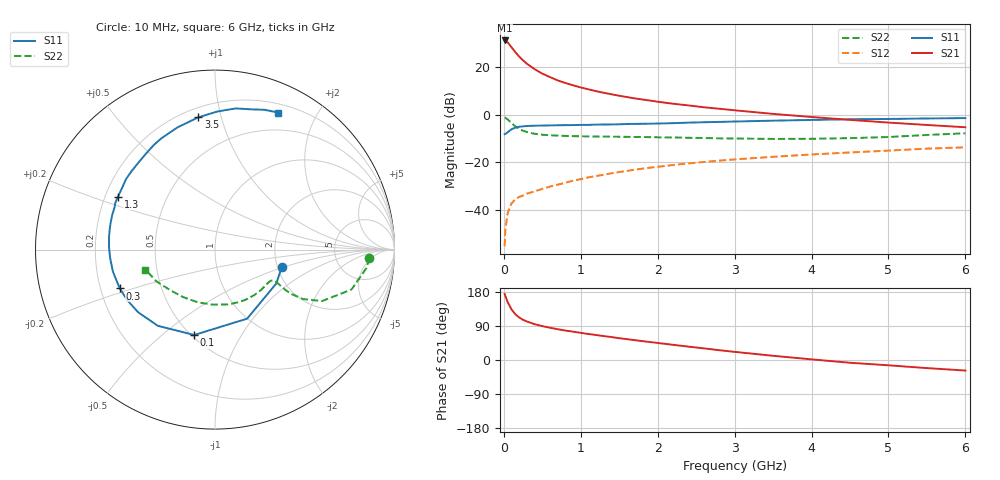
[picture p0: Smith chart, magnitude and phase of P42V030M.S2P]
! SIEMENS Small Signal Semiconductors
! BFP182
! Si NPN RF Bipolar Junction Transistor in SOT143
! VCE = 2 V  IC = 30 mA
! Common Emitter S-Parameters:  March  1996
# GHz  S  MA  R  50
!  f  S11  S21  S12  S22
! GHz  MAG  ANG  MAG  ANG  MAG  ANG  MAG  ANG
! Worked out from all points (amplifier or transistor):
!   36 points, 10 MHz to 6 GHz, reference 50 ohm
!   highest |S21| = 31.2 dB at 10 MHz (marker M1)
!   |S21| within 3 dB of that: start of sweep to 102.9 MHz
!   unconditionally stable (mu >= 1): start of sweep to 17.58 MHz; 309.4 MHz to end of sweep
!   at 250 MHz: K = 0.90, MSG = 28.4 dB, |S12| = -34.1 dB
!   at 1.4 GHz: K = 1.63, MAG = 12.0 dB, |S12| = -24.7 dB
!   at 6 GHz: K = 1.15, MAG = 1.8 dB, |S12| = -13.8 dB
!   S11 on the Smith chart (normalised r, x): 10 MHz: 2.11, -0.48; 100 MHz: 0.52, -0.65; 300 MHz: 0.28, -0.18; 1.3 GHz: 0.25, +0.24; 3.5 GHz: 0.26, +0.85; 6 GHz: 0.29, +1.52
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0.01  0.3846 -14.6  36.18 174.2  0.0017 75.7  0.8603 -3.1
0.02  0.3903 -28.9  35.97 168.9  0.0038 73.8  0.8513 -6.8
0.05  0.4244 -65.1  33.08 152.7  0.0085 71.5  0.7923 -16.3
0.1  0.4897 -103.7  25.97 133.4  0.0135 54.7  0.6617 -25.7
0.15  0.5308 -126.9  20.45 120.6  0.0166 48.1  0.5628 -29.3
0.2  0.5528 -140.9  16.56 112.1  0.0185 46.9  0.4966 -30.1
0.25  0.5647 -150.4  13.76 106.1  0.0198 47.6  0.4551 -29.9
0.3  0.5732 -157.8  11.72 101.6  0.0217 47.6  0.4274 -29.1
0.4  0.582 -168.0  8.989 94.5  0.0241 49.6  0.3936 -28.1
0.5  0.5859 -175.2  7.256 89.4  0.0273 50.9  0.3756 -27.8
0.6  0.5906 178.9  6.129 85.1  0.0305 53.5  0.3665 -28.0
0.7  0.5946 173.5  5.224 81.2  0.0334 55.4  0.3595 -28.7
0.8  0.5973 169.3  4.61 77.7  0.0367 55.8  0.3544 -29.6
1.1  0.6062 157.8  3.386 68.6  0.0477 57.4  0.3465 -33.9
1.3  0.616 151.3  2.862 63.1  0.0542 57.4  0.3433 -37.3
1.7  0.6355 138.7  2.187 52.4  0.069 56.1  0.3375 -45.2
2.2  0.6581 125.9  1.688 40.0  0.0866 52.9  0.329 -56.4
2.8  0.6993 111.0  1.322 25.9  0.107 47.6  0.3158 -71.7
3.5  0.7427 97.2  1.032 11.1  0.129 41.2  0.3068 -92.5
4.5  0.7948 81.7  0.772 -7.3  0.1592 32.0  0.3185 -123.7
5.5  0.8263 70.5  0.603 -21.4  0.1917 22.8  0.3715 -151.6
6  0.8411 65.2  0.54 -27.8  0.2043 17.2  0.4031 -164.0
